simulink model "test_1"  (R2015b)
settings: Solver=VariableStepAuto  StartTime=0.0  StopTime=200.0  RelTol=1e-3
undefined symbols (not defined in the file or in its folder): fir1
libraries: simulink x1, dspsigops x1, dspstat3 x1

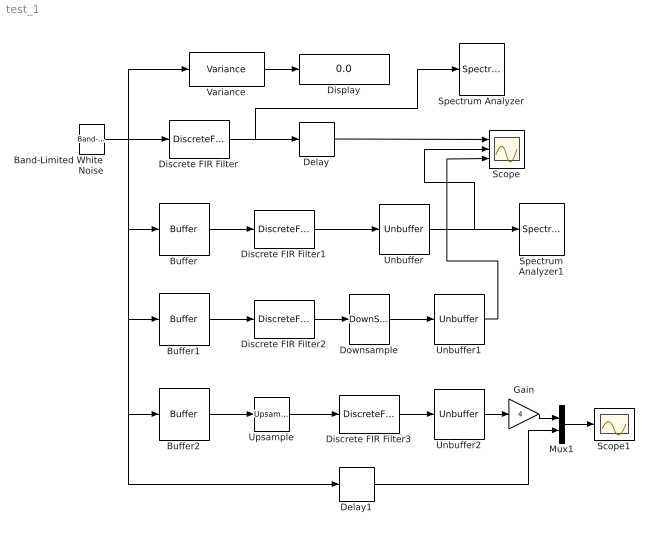
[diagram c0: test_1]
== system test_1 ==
  Band-Limited White Noise : simulink/Sources/Band-Limited White Noise  Cov=[0.01]  Ts=0.01  seed=[23341]
  Buffer : Buffer  N=512*4  TreatMby1Signals=One channel  OutputFrames=off
  Buffer1 : Buffer  N=512*4  TreatMby1Signals=One channel  OutputFrames=off
  Buffer2 : Buffer  N=512*4  TreatMby1Signals=One channel  OutputFrames=off
  Delay : Delay  DelayLength=2048
  Delay1 : Delay  DelayLength=2048+8
  Discrete FIR Filter : DiscreteFir  Coefficients=fir1(64, 0.5);
  Discrete FIR Filter1 : DiscreteFir  Coefficients=fir1(64, 0.5);  InputProcessing=Columns as channels (frame based)
  Discrete FIR Filter2 : DiscreteFir  Coefficients=fir1(64, 0.5);  InputProcessing=Columns as channels (frame based)
  Discrete FIR Filter3 : DiscreteFir  Coefficients=fir1(64, 0.25);  InputProcessing=Columns as channels (frame based)
  Display : Display
  Downsample : DownSample  N=4  RateOptions=Allow multirate processing
  Gain : Gain  Gain=4
  Mux1 : Mux  Inputs=2
  Scope : Scope  NumInputPorts=3
  Scope1 : Scope
  Spectrum Analyzer : SpectrumAnalyzer
  Spectrum Analyzer1 : SpectrumAnalyzer
  Unbuffer : Unbuffer  SampleBasedProcessing=Same as frame based
  Unbuffer1 : Unbuffer  SampleBasedProcessing=Same as frame based
  Unbuffer2 : Unbuffer  SampleBasedProcessing=Same as frame based
  Upsample : dspsigops/Upsample  N=4  phase=0  InputProcessing=Columns as channels (frame based)  RateOptions=Allow multirate processing  ic=0  mode=Unused parameter value
  Variance : dspstat3/Variance  run=on  reset_popup=None  directionMode=Each column  dimension=1  roiEnable=off  roiType=Rectangles  roiPortion=Entire ROI  roiOutput=Individual statistics for each ROI  roiFlag=off  roundingMode=Floor  overflowMode=off
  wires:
  Band-Limited White Noise/1 -> Variance/1, Discrete FIR Filter/1, Buffer/1, Buffer1/1, Delay1/1, Buffer2/1
  Discrete FIR Filter1/1 -> Unbuffer/1
  Unbuffer/1 -> Scope/2, Spectrum Analyzer1/1
  Delay/1 -> Scope/1
  Variance/1 -> Display/1
  Buffer/1 -> Discrete FIR Filter1/1
  Buffer1/1 -> Discrete FIR Filter2/1
  Discrete FIR Filter2/1 -> Downsample/1
  Downsample/1 -> Unbuffer1/1
  Unbuffer1/1 -> Scope/3
  Discrete FIR Filter3/1 -> Unbuffer2/1
  Buffer2/1 -> Upsample/1
  Upsample/1 -> Discrete FIR Filter3/1
  Unbuffer2/1 -> Gain/1
  Discrete FIR Filter/1 -> Delay/1, Spectrum Analyzer/1
  Gain/1 -> Mux1/1
  Delay1/1 -> Mux1/2
  Mux1/1 -> Scope1/1
